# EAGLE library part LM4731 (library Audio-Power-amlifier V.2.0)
LM4731 Stereo 25W Audio Power Amplifier with Mute and Standby Modes
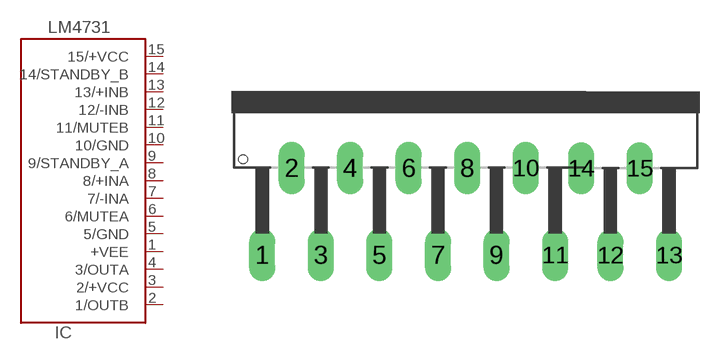
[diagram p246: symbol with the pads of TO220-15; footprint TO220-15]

Designator prefix IC

## LM4731  [TO220-15]
1  +VEE  pwr
2  1/OUTB  out
3  2/+VCC  pwr
4  3/OUTA  out
5  5/GND  pwr
6  6/MUTEA  in
7  7/-INA  in
8  8/+INA  in
9  9/STANDBY_A  in
10  10/GND  pwr
11  11/MUTEB  in
12  12/-INB  in
13  13/+INB  in
14  14/STANDBY_B  in
15  15/+VCC  pwr

## Footprint TO220-15 (pad centres in mm)
drill 1.016 long: 1 0.381,1.905; 2 2.083,6.96; 3 3.785,1.905; 4 5.486,6.96; 5 7.188,1.905; 6 8.89,6.96; 7 10.592,1.905; 8 12.294,6.96; 9 13.995,1.905; 10 15.697,6.96; 11 17.399,1.905; 12 20.615,1.895; 13 24.019,1.895; 14 18.914,6.95; 15 22.317,6.95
